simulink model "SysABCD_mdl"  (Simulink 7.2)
settings: Solver=ode45  StartTime=0.0  StopTime=10.0  RelTol=1e-3
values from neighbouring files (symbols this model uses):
  A = [0 1; -k/M -h/M]    [SistemaMassaMolla.m]
  B = [0; 1/M]    [SistemaMassaMolla.m]
  C = [1 0]    [SistemaMassaMolla.m]
  D = [0]    [SistemaMassaMolla.m]
  X0 = [0;0]    [SistemaMassaMolla.m]

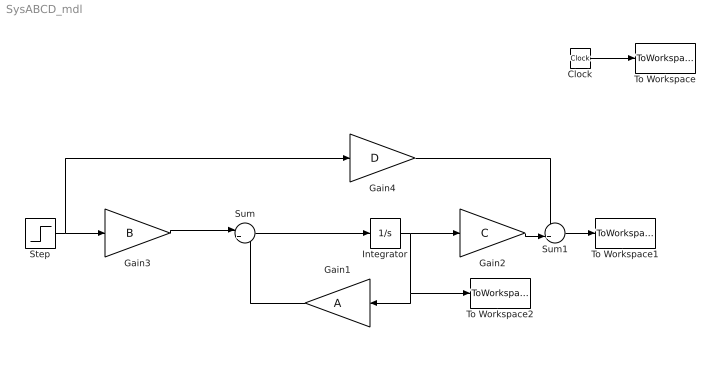
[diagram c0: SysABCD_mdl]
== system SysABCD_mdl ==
  Clock : Clock
  Gain1 : Gain  Orientation=left  Gain=A  Multiplication=Matrix(K*u)  ParameterDataType=sfix(16)  ParameterScaling=2^0  OutDataType=sfix(16)  OutScaling=2^0
  Gain2 : Gain  Gain=C  Multiplication=Matrix(K*u)  ParameterDataType=sfix(16)  ParameterScaling=2^0  OutDataType=sfix(16)  OutScaling=2^0
  Gain3 : Gain  Gain=B  Multiplication=Matrix(K*u)  ParameterDataType=sfix(16)  ParameterScaling=2^0  OutDataType=sfix(16)  OutScaling=2^0
  Gain4 : Gain  Gain=D  Multiplication=Matrix(K*u)  ParameterDataType=sfix(16)  ParameterScaling=2^0  OutDataType=sfix(16)  OutScaling=2^0
  Integrator : Integrator  InitialCondition=X0
  Step : Step  SampleTime=0
  Sum : Sum  Inputs=|++  OutDataType=sfix(16)  OutScaling=2^0
  Sum1 : Sum  Inputs=++|  OutDataType=sfix(16)  OutScaling=2^0
  To Workspace : ToWorkspace  VariableName=time  SampleTime=-1  SaveFormat=Array
  To Workspace1 : ToWorkspace  VariableName=y  SampleTime=-1  SaveFormat=Array
  To Workspace2 : ToWorkspace  VariableName=x  SampleTime=-1  SaveFormat=Array
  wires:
  Gain3/1 -> Sum/1
  Gain1/1 -> Sum/2
  Sum/1 -> Integrator/1
  Integrator/1 -> Gain2/1, Gain1/1, To Workspace2/1
  Step/1 -> Gain3/1, Gain4/1
  Clock/1 -> To Workspace/1
  Gain2/1 -> Sum1/2
  Sum1/1 -> To Workspace1/1
  Gain4/1 -> Sum1/1
